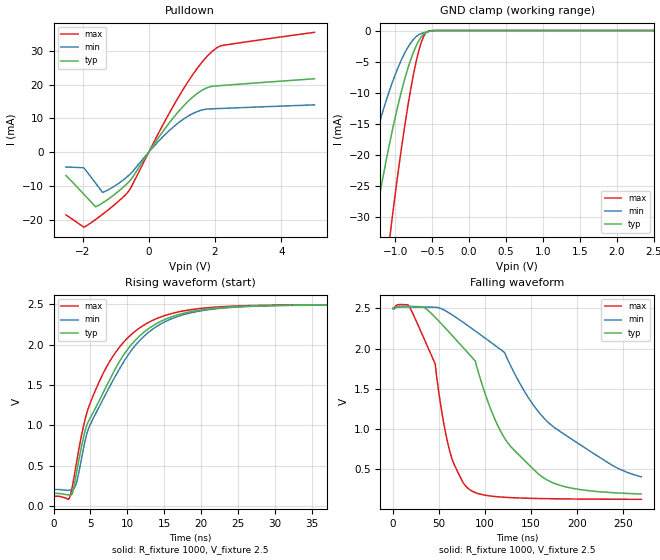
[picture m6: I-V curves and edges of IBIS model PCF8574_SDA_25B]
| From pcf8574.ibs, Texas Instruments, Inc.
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[Model]   PCF8574_SDA_25B
Model_type  I/O_open_drain
Vinl=.75
Vinh=1.75
Enable   Active-Low
Vref =   2.5
Rref =   4700
Cref =   10p
Vmeas =   1.25
| variable   typ   min   max
C_comp   1.93pF   1.42pF   2.31pF
| C_pulldown   1.26pF   1.09pF   1.51pF
| C_tri-state   1.93pF   1.42pF   2.31pF
[Temperature Range]   40   100   -40
| Ambient temperature   25   85   -40
[Voltage range]   2.5   2.5   2.5
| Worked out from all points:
|   slope of the pulldown table from 0 to 0.375 V, typ, clamps not added: 69.1 ohm
|   GND clamp passes 1 mA (typ) near -0.65 V on its own axis
|   rising waveform, R_fixture 1000, V_fixture 2.5: 20-80 % time 7.28ns typ, 7.59ns min, 6.2ns max; typ from 0.158 V to 2.5 V
|   falling waveform, R_fixture 1000, V_fixture 2.5: 20-80 % time 64.7ns typ, 94.7ns min, 27.5ns max; typ from 2.5 V to 0.191 V
[GND Clamp]
| PCF8574_SDA_25B
|   Voltage   I(typ)   I(min)   I(max)
-2.5V     -148.9mA   -106.8mA   -225.5mA
-1.555V   -51.46mA   -33.82mA   -88.02mA
-1.515V   -48.32mA   -31.06mA   -83.03mA
-1.395V   -39.26mA   -23.03mA   -68.46mA
-1.285V   -31.44mA   -17.9mA    -55.72mA
-1.065V   -17.53mA   -9.236mA   -32.48mA
-830mV    -6.152mA   -2.746mA   -12.26mA
-740mV    -3.121mA   -1.268mA   -6.33mA
-670mV    -1.43mA    -608.2uA   -2.812mA
-600mV    -446.9uA   -315.3uA   -632.8uA
-515mV    -65.33uA   -72.81uA   -12.92uA
2.5V      277.9pA    456.8pA    79.62pA
[Pulldown]
| PCF8574_SDA_25B
|   Voltage   I(typ)   I(min)   I(max)
-2.5V     -6.916mA   -4.415mA   -18.56mA
-1.96V    -12.45mA   -4.667mA   -22.21mA
-1.61V    -16.15mA   -9.118mA   -19.98mA
-1.44V    -15.31mA   -11.34mA   -18.75mA
-1.2V     -13.76mA   -11.02mA   -16.91mA
-585mV    -8.619mA   -6.689mA   -11.2mA
335mV     4.872mA    3.643mA    6.395mA
970mV     12.83mA    9.249mA    17.51mA
1.53V     17.85mA    12.26mA    25.7mA
1.995V    19.58mA    12.87mA    30.49mA
2.24V     19.77mA    12.97mA    31.65mA
5V        21.73mA    14.01mA    35.49mA
[Ramp]
| PCF8574_SDA_25B
| variable   typ   min   max
dV/dt_r   1.42/7.27E-09   1.38/7.58E-09   1.45/6.18E-09
dV/dt_f   1.40/6.59E-08   1.27/9.61E-08   1.46/2.87E-08
R_load = 1000
[Rising Waveform]
| PCF8574_SDA_25B
R_fixture =   1000
C_fixture =   0
L_fixture =   0
V_fixture =   2.5
V_fixture_min = 2.5
V_fixture_max = 2.5
|   Time   V(typ)   V(min)   V(max)
0s        157.7mV    206.4mV    122.7mV
2ns       140.9mV    196.3mV    84.45mV
2.5ns     149.8mV    199.2mV    221.9mV
3.1ns     410.3mV    288.1mV    535.8mV
4.7ns     1.046V     950.6mV    1.212V
6.8ns     1.421V     1.342V     1.66V
9ns       1.804V     1.713V     1.979V
13.7ns    2.25V      2.212V     2.315V
20.5ns    2.44V      2.429V     2.457V
269.9ns   2.5V       2.5V       2.5V
[Falling Waveform]
| PCF8574_SDA_25B
R_fixture =   1000
C_fixture =   0
L_fixture =   0
V_fixture =   2.5
V_fixture_min = 2.5
V_fixture_max = 2.5
|   Time   V(typ)   V(min)   V(max)
0s        2.5V       2.5V       2.5V
17.3ns    2.526V     2.519V     2.535V
46ns      2.39V      2.515V     1.811V
53.7ns    2.297V     2.492V     1.177V
61.9ns    2.195V     2.439V     721.8mV
82.7ns    1.934V     2.277V     251.4mV
89.6ns    1.846V     2.22V      207.9mV
119.6ns   920.1mV    1.968V     151.4mV
159.4ns   428.5mV    1.198V     134.4mV
269.9ns   191mV      404.1mV    124.5mV
